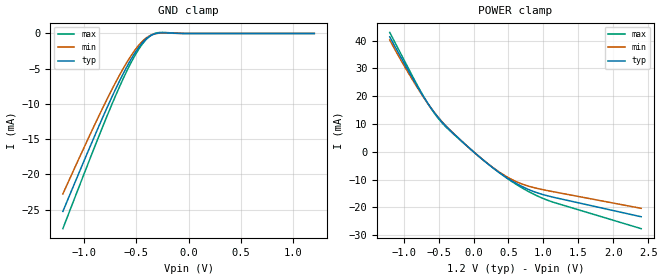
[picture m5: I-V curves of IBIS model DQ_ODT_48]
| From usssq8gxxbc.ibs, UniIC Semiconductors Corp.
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|   Model DQ_ODT_48
[Model] DQ_ODT_48
Model_type Input
Polarity   Non-Inverting
Enable   Active-High
Vinl =  8.300E-01
Vinh =  9.700E-01
C_comp   6.947E-13   6.927E-13   6.952E-13
C_comp_power_clamp   2.710E-13   2.694E-13   2.743E-13
C_comp_gnd_clamp   4.063E-13   4.053E-13   4.098E-13
[Model Spec]
Vinh   9.700E-01   9.250E-01   1.015E+00
Vinl   8.300E-01   7.850E-01   8.750E-01
[Temperature Range]   4.500E+01   9.500E+01   0.000E+00
[Voltage Range]   1.200E+00   1.140E+00   1.260E+00
[C Comp Corner]
C_comp_power_clamp   2.710E-13   2.743E-13   2.694E-13
C_comp_gnd_clamp   4.063E-13   4.053E-13   4.098E-13
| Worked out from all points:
|   GND clamp passes 1 mA (typ) near -0.42 V on its own axis
|   POWER clamp passes 1 mA (typ) near -0.04 V on its own axis
[GND_clamp]
|Voltage   I(typ)   I(min)   I(max)
-1.2V     -25.25mA   -22.78mA   -27.69mA
-875mV    -13.8mA    -12.29mA   -15.28mA
-750mV    -9.605mA   -8.487mA   -10.7mA
-650mV    -6.471mA   -5.667mA   -7.258mA
-575mV    -4.342mA   -3.761mA   -4.895mA
-500mV    -2.497mA   -2.13mA    -2.824mA
-425mV    -1.067mA   -892.7uA   -1.198mA
-375mV    -421.9uA   -355.4uA   -450.2uA
-325mV    -57.46uA   -63.78uA   -13.32uA
-250mV    84.35uA    53.31uA    150.7uA
-25mV     0A         0A         0A
1.2V      0A         0A         0A
[POWER_clamp]
|Voltage   I(typ)   I(min)   I(max)
-1.2V     41.39mA    40.31mA    42.99mA
-1V       32.2mA     31.26mA    33.31mA
-775mV    22.25mA    21.93mA    22.59mA
-650mV    17.26mA    17.21mA    17.24mA
-525mV    12.93mA    13.02mA    12.67mA
-375mV    8.717mA    8.811mA    8.455mA
-75mV     1.678mA    1.681mA    1.642mA
175mV     -3.735mA   -3.693mA   -3.7mA
375mV     -7.597mA   -7.389mA   -7.63mA
675mV     -12.25mA   -11.41mA   -12.71mA
1.025V    -15.62mA   -13.8mA    -17.1mA
2.4V      -23.39mA   -20.36mA   -27.67mA
